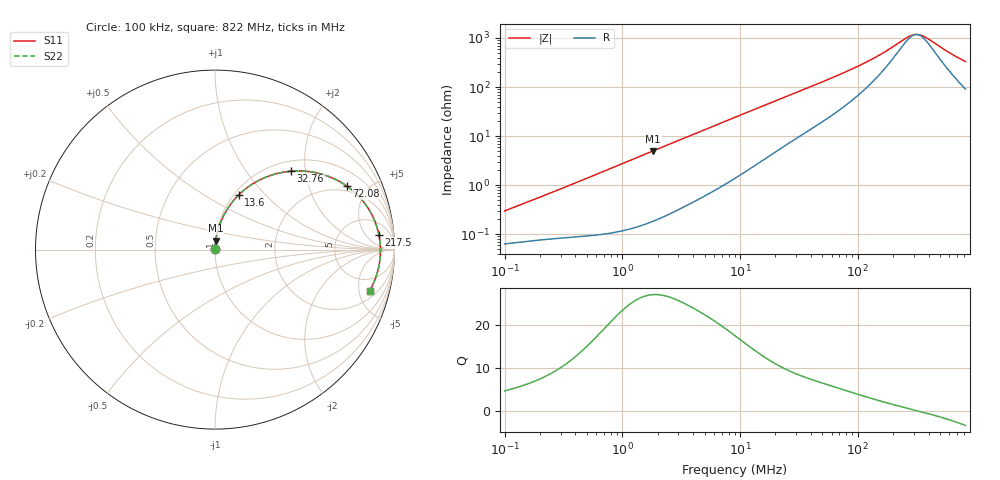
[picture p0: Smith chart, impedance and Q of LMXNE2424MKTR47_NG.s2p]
! LMXNE2424MKTR47_NG  S-PARAMETER MODEL  ( General Type )
! Model Generated by TAIYO YUDEN Corporation (http://www.ty-top.com)
! Version 1.0
! TAIYO YUDEN Control No. 191023NI43SB-FBB
! Copyright(c) 2019 TAIYO YUDEN CO.,LTD. All Rights Reserved.
! Product Description (link to TY-COMPAS)
! https://ds.yuden.co.jp/TYCOMPAS/or/detail?pn=LMXNE2424MKTR47NNG&u=M
! Products Name : Inductors
! Characteristics :
!  Inductance : 0.47 uH , SRF(min) : 180 MHz , DC Resistance(max) : 0.06 Ohm
!  Rated Current : Saturation :2900 mA , Temp Rise : 2100 mA
!  Case Size : 2.4 x 2.4 / 0.094 x 0.094 [mm/inch] , Thickness : 1.2 / 0.047 [mm/inch]
!  (Conditions: Temperature = 25 degC , DC Bias Current/Voltage = 0A / 0V)
! External Node Assignments :
!  1  o---GGG---o  2
! GND o---------o GND
! Frequency Range : 0.1MHz  -  821.96004MHz  [ 402 STEP ]
# MHz S RI R 50
! Freq[MHz].  S11 Real  S11 Imag  S21 Real  S21 Imag  S12 Real  S12 Imag  S22 Real  S22 Imag
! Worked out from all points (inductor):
!   401 points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, 100 kHz to 822 MHz, reference 50 ohm
!   read as one part in series: L = 459 nH near 104.6 kHz
!   highest Q = 27.1 at 1.83 MHz (marker M1), where L = 435 nH
!   self-resonance near 314.8 MHz
!   S11 on the Smith chart (normalised r, x): 100 kHz: 1.00, +0.01; 13.6 MHz: 1.05, +0.72; 32.76 MHz: 1.20, +1.67; 72.08 MHz: 1.72, +3.63; 217.5 MHz: 11, +12; 822 MHz: 2.83, -6.35
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0.1  0.000642 0.00291  0.9994 -0.00291  0.9994 -0.00291  0.000642 0.00291
0.452624  0.00105 0.0125  0.9989 -0.0125  0.9989 -0.0125  0.00105 0.0125
1.830372  0.00432 0.0497  0.9957 -0.0497  0.9957 -0.0497  0.00432 0.0497
2.048684  0.00515 0.0555  0.9948 -0.0555  0.9948 -0.0555  0.00515 0.0555
4.611174  0.0203 0.1211  0.9797 -0.1211  0.9797 -0.1211  0.0203 0.1211
9.272834  0.0691 0.2264  0.9309 -0.2264  0.9309 -0.2264  0.0691 0.2264
13.60171  0.1312 0.3037  0.8688 -0.3037  0.8688 -0.3037  0.1312 0.3037
20.40619  0.241 0.384  0.759 -0.384  0.759 -0.384  0.241 0.384
32.75605  0.4237 0.4368  0.5763 -0.4368  0.5763 -0.4368  0.4237 0.4368
41.03579  0.5204 0.4351  0.4796 -0.4351  0.4796 -0.4351  0.5204 0.4351
53.77846  0.632 0.4079  0.368 -0.4079  0.368 -0.4079  0.632 0.4079
72.08436  0.7356 0.3531  0.2644 -0.3531  0.2644 -0.3531  0.7356 0.3531
118.3471  0.8529 0.2309  0.1471 -0.2309  0.1471 -0.2309  0.8529 0.2309
185.7378  0.904 0.1195  0.096 -0.1195  0.096 -0.1195  0.904 0.1195
217.4754  0.9131 0.0828  0.0869 -0.0828  0.0869 -0.0828  0.9131 0.0828
254.6362  0.9189 0.0471  0.0811 -0.0471  0.0811 -0.0471  0.9189 0.0471
285.0071  0.9211 0.022  0.0789 -0.022  0.0789 -0.022  0.9211 0.022
311.892  0.9219 0.00204  0.0781 -0.00204  0.0781 -0.00204  0.9219 0.00204
341.3129  0.9217 -0.018  0.0783 0.018  0.0783 0.018  0.9217 -0.018
390.7289  0.9198 -0.0482  0.0802 0.0482  0.0802 0.0482  0.9198 -0.0482
627.1987  0.894 -0.1605  0.106 0.1605  0.106 0.1605  0.894 -0.1605
821.96  0.8609 -0.231  0.1391 0.231  0.1391 0.231  0.8609 -0.231
